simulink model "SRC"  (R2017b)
settings: Solver=ode15s  StartTime=0.0  StopTime=6000  MaxStep=0.1  RelTol=1e-5
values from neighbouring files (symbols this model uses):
  d = Tin_c(i)    [ActiveConstraints.m]    (also in Main.m = 293.15)
  Kc = -0.06    [Main.m]
  N = 10    [ActiveConstraints.m]    (also in Main.m; SRC_ODE.m = p(8))
  p = [rho_c; rho_h; Tin_h; U; A; cp_c; cp_h;N;F_c_max;F_h_max]    [ActiveConstraints.m]    (also in Main.m)
  tauI = 80    [Main.m]
  ThSP = x0(end)    [ActiveConstraints.m]    (also in Main.m)
  x0 = [Tc0; Th0]    [ActiveConstraints.m]    (also in Main.m; col_obj.m = 0.5*ones(1,82)'; Simulate1Col.m = x; Simulate1Col_OL.m = x)
undefined symbols (not defined in the file or in its folder): SRC_ODE
libraries: simulink x1

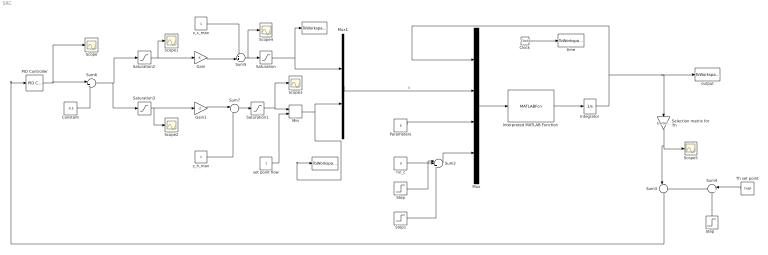
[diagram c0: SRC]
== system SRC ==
  " " : ToWorkspace  VariableName=u1  SampleTime=-1
  "  " : ToWorkspace  VariableName=u2  SampleTime=-1
  Clock : Clock
  Constant : Constant  Value=-0.5
  Gain : Gain
  Gain1 : Gain  Gain=-2
  Integrator : Integrator  InitialCondition=x0'
  Interpreted MATLAB Function : MATLABFcn  MATLABFcn=SRC_ODE(u(1:20),u(21:22),u(23:32),u(33))  OutputDimensions=20  Output1D=off
  Min : MinMax  Inputs=2
  Mux : Mux
  Mux1 : Mux  Inputs=2
  PID Controller : simulink/Continuous/PID Controller  Controller=PI  TimeDomain=Continuous-time  SampleTime=-1  IntegratorMethod=Forward Euler  FilterMethod=Forward Euler  Form=Parallel  UseFilter=on  ControllerParametersSource=internal  P=Kc  I=Kc/tauI  D=0  N=100  InitialConditionSource=internal  InitialConditionForIntegrator=0  InitialConditionForFilter=0  ExternalReset=none  IgnoreLimit=on  ZeroCross=off  LimitOutput=off  UpperSaturationLimit=1  LowerSaturationLimit=0  LinearizeAsGain=on  AntiWindupMode=back-calculation  Kb=1  TrackingMode=off  Kt=1  PParamMin=[]  PParamMax=[]  IParamMin=[]  IParamMax=[]  DParamMin=[]  DParamMax=[]  NParamMin=[]  NParamMax=[]  KbParamMin=[]  KbParamMax=[]  KtParamMin=[]  KtParamMax=[]  POutMin=[]  POutMax=[]  IOutMin=[]  IOutMax=[]  DOutMin=[]  DOutMax=[]  NOutMin=[]  NOutMax=[]  KbOutMin=[]  KbOutMax=[]  KtOutMin=[]  KtOutMax=[]  IntegratorOutMin=[]  IntegratorOutMax=[]  FilterOutMin=[]  FilterOutMax=[]  SumOutMin=[]  SumOutMax=[]  SumI1OutMin=[]  SumI1OutMax=[]  SumI2OutMin=[]  SumI2OutMax=[]  SumI3OutMin=[]  SumI3OutMax=[]  SumDOutMin=[]  SumDOutMax=[]  SaturationOutMin=[]  SaturationOutMax=[]  IntegratorContinuousStateAttributes=''  IntegratorStateMustResolveToSignalObject=off  IntegratorRTWStateStorageClass=Auto  FilterContinuousStateAttributes=''  FilterStateMustResolveToSignalObject=off  FilterRTWStateStorageClass=Auto  DifferentiatorICPrevScaledInput=0  DifferentiatorOutMin=[]  DifferentiatorOutMax=[]  InitialConditionSetting=State (most efficient)  FilterDiffOutCoefMin=[]  FilterDiffOutCoefMax=[]  SumDenOutMin=[]  SumDenOutMax=[]  SumNumOutMin=[]  SumNumOutMax=[]  ReciprocalOutMin=[]  ReciprocalOutMax=[]  DivideOutMin=[]  DivideOutMax=[]  TunerSelectOption=Transfer Function Based (PID Tuner App)
  Parameters : Constant  Value=p
  Saturation : Saturate  UpperLimit=1  LowerLimit=0
  Saturation1 : Saturate  UpperLimit=1  LowerLimit=0
  Saturation2 : Saturate  UpperLimit=0  LowerLimit=-100
  Saturation3 : Saturate  UpperLimit=100  LowerLimit=0
  Scope{,1..5} (6 alike) : Scope
  Selection matrix for Th : Gain  Gain=[zeros(1,2*N-1),1]  Multiplication=Matrix(K*u)
  Step : Step  Time=200  After=2  SampleTime=0
  "Step   " : Step  Time=50  After=0  SampleTime=0
  Step1 : Step  Time=2000  After=4  SampleTime=0
  Sum2 : Sum  Inputs=|+++
  Sum3 : Sum  Inputs=|-+
  Sum4 : Sum  Inputs=|++
  Sum5 : Sum  Inputs=++|
  Sum6 : Sum  Inputs=|++
  Sum7 : Sum  Inputs=|++
  Th set point : Constant  Value=ThSP
  Tin_c : Constant  Value=d
  output : ToWorkspace  VariableName=y  SampleTime=-1
  set point flow : Constant
  time : ToWorkspace  VariableName=t  SampleTime=-1
  z_c_max : Constant
  z_h_max : Constant
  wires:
  Interpreted MATLAB Function/1 -> Integrator/1
  Integrator/1 -> Mux/1, Selection matrix for Th/1, output/1
  Mux/1 -> Interpreted MATLAB Function/1
  Clock/1 -> time/1
  Mux1/1 -> Mux/2  "u"
  Parameters/1 -> Mux/3
  Tin_c/1 -> Sum2/1
  Step/1 -> Sum2/2
  Sum2/1 -> Mux/4
  Sum4/1 -> Sum3/2
  "Step   "/1 -> Sum4/2
  Th set point/1 -> Sum4/1
  Sum3/1 -> PID Controller/1
  z_h_max/1 -> Sum7/2
  Saturation/1 -> Mux1/1, " "/1
  Sum5/1 -> Scope4/1, Saturation/1
  Saturation1/1 -> Scope3/1, Min/1
  Selection matrix for Th/1 -> Sum3/1, Scope5/1
  Saturation2/1 -> Scope1/1, Gain/1
  Saturation3/1 -> Scope2/1, Gain1/1
  Gain/1 -> Sum5/2
  Gain1/1 -> Sum7/1
  Sum7/1 -> Saturation1/1
  PID Controller/1 -> Sum6/1, Scope/1
  Sum6/1 -> Saturation3/1, Saturation2/1
  Constant/1 -> Sum6/2
  z_c_max/1 -> Sum5/1
  set point flow/1 -> Min/2
  Min/1 -> "  "/1, Mux1/2
  Step1/1 -> Sum2/3
